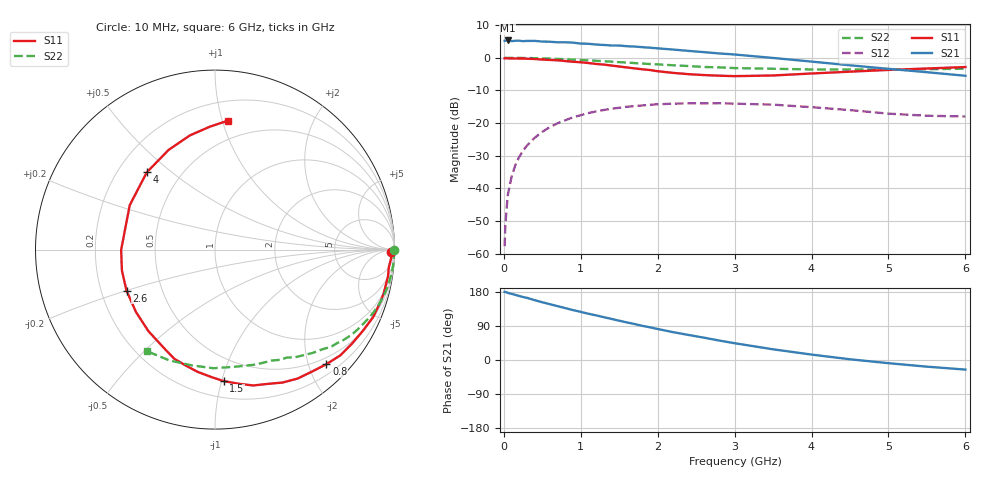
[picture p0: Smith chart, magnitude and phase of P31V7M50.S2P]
! SIEMENS Small Signal Semiconductors
! BFP181
! Si NPN RF Bipolar Junction Transistor in SOT143
! VCE = 1.75 V  IC = 0.5 mA
! Common Emitter S-Parameters:  March  1996
# GHz  S  MA  R  50
!  f  S11  S21  S12  S22
! GHz  MAG  ANG  MAG  ANG  MAG  ANG  MAG  ANG
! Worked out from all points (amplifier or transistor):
!   36 points, 10 MHz to 6 GHz, reference 50 ohm
!   highest |S21| = 5.3 dB at 50 MHz (marker M1)
!   |S21| within 3 dB of that: start of sweep to 2.304 GHz
!   unconditionally stable (mu >= 1): 3.712 GHz to end of sweep
!   at 250 MHz: K = 0.08, MSG = 16.8 dB, |S12| = -28.4 dB
!   at 1.4 GHz: K = 0.44, MSG = 9.7 dB, |S12| = -15.6 dB
!   at 6 GHz: K = 1.47, MAG = 2.2 dB, |S12| = -18.0 dB
!   S11 on the Smith chart (normalised r, x): 10 MHz: 69, -38; 800 MHz: 0.38, -2.32; 1.5 GHz: 0.32, -1.02; 2.6 GHz: 0.31, -0.20; 4 GHz: 0.32, +0.41; 6 GHz: 0.35, +1.04
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0.01  0.9782 -0.7  1.819 179.8  0.0013 89.3  0.9996 -0.2
0.02  0.9831 -1.0  1.831 179.6  0.0028 84.7  0.9993 -0.6
0.05  0.9828 -2.7  1.842 177.3  0.0077 90.5  0.998 -1.4
0.1  0.9734 -5.8  1.796 174.6  0.0149 85.4  0.9977 -2.8
0.15  0.9754 -8.8  1.823 171.8  0.0229 83.5  0.9966 -4.1
0.25  0.971 -14.5  1.795 166.2  0.0379 79.9  0.9928 -7.1
0.4  0.9579 -23.2  1.816 157.9  0.0594 74.0  0.9861 -11.2
0.5  0.9397 -28.9  1.771 152.4  0.0733 69.1  0.9789 -13.9
0.8  0.8905 -45.8  1.728 136.9  0.1107 57.9  0.9496 -21.7
0.9  0.8686 -51.4  1.705 131.6  0.1224 53.8  0.9368 -24.2
1.1  0.8308 -63.1  1.638 122.0  0.1423 46.6  0.912 -29.0
1.5  0.7344 -86.2  1.54 103.7  0.1716 33.6  0.8564 -37.5
1.9  0.6492 -110.4  1.427 86.2  0.1902 22.2  0.8023 -45.0
2.2  0.5867 -129.2  1.336 73.5  0.1979 14.6  0.7673 -50.1
2.6  0.5434 -155.1  1.22 59.0  0.2 5.9  0.7224 -56.4
3  0.523 -179.8  1.122 44.3  0.1981 -2.7  0.6948 -62.8
3.5  0.5356 152.5  0.994 28.2  0.1915 -10.7  0.679 -70.7
4  0.5744 131.4  0.874 14.3  0.175 -17.1  0.6623 -80.2
4.5  0.6127 114.9  0.767 1.9  0.1579 -21.6  0.661 -90.7
5  0.6515 102.4  0.677 -8.4  0.1393 -22.0  0.6579 -101.5
5.5  0.685 92.5  0.601 -17.6  0.1294 -18.5  0.6678 -112.5
6  0.7213 84.4  0.53 -25.3  0.1262 -14.4  0.6807 -123.7
